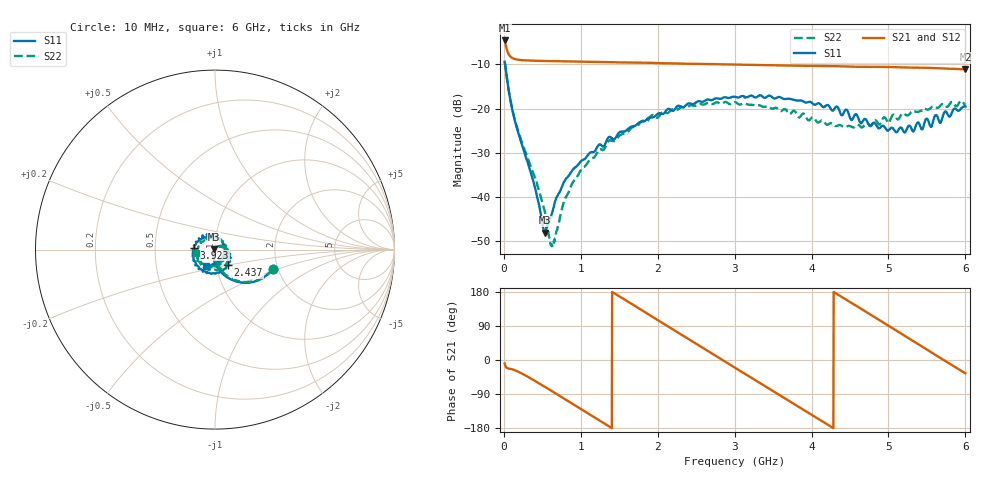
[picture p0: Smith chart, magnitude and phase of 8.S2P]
!Agilent Technologies,E5071C,MY46316741,A.11.02
!Date: Thu Jul 30 16:12:56 2020
!Data & Calibration Information:
!Freq	S11:SOLT4(ON)	S21:SOLT4(ON)	S12:SOLT4(ON)	S22:SOLT4(ON)
!PortZ  Port1:50+j0  Port2:50+j0
!Above PortZ is port z conversion or system Z0 setting when saving the data.
!When reading, reference impedance value at option line is always used.
# Hz S dB R 50
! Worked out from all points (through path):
!   1561 points, 10 MHz to 6 GHz, reference 50 ohm
!   highest |S21| = -4.55 dB at 10 MHz (marker M1); lowest = -11.1 dB at 6 GHz (marker M2)
!   group delay of S21, straight-line fit = 347 ps
!   lowest |S11| = -48.2 dB at 536 MHz (marker M3), VSWR 1.01, Z = 49.6 + j0.164 ohm
!   |S11| at or under -10 dB: 16.33 MHz to end of sweep
!   |S22| runs from -51.2 to -9.3 dB; largest |S21 - S12| = 0.0045
!   S11 on the Smith chart (normalised r, x): 10 MHz: 1.88, -0.46; 2.437 GHz: 1.14, -0.20; 3.923 GHz: 0.79, +0.02; 6 GHz: 0.89, -0.17
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1e7  -9.37 -18.6  -4.55 -9.1  -4.55 -9.1  -9.34 -18.2
5.991667e7  -15.52 -66.5  -7.59 -22.5  -7.59 -22.5  -15.48 -63.7
1.136731e8  -20.59 -83.8  -8.57 -24.9  -8.56 -24.9  -20.48 -78.3
3.786154e8  -36.22 -125.3  -9.15 -52.1  -9.14 -52.2  -34.53 -95.8
5.360449e8  -48.19 154.9  -9.21 -71.1  -9.21 -71.2  -43.60 -84.3
5.974808e8  -45.26 108.7  -9.23 -78.7  -9.23 -78.8  -50.08 -60.3
6.358782e8  -43.14 88.3  -9.25 -83.4  -9.24 -83.5  -50.97 -23.1
7.894679e8  -36.49 62.1  -9.29 -102.5  -9.29 -102.7  -40.59 42.0
1.012173e9  -31.80 46.9  -9.35 -130.4  -9.35 -130.6  -33.70 41.9
1.488301e9  -25.67 16.2  -9.53 169.7  -9.52 169.4  -26.42 15.0
2.006667e9  -21.13 -17.1  -9.69 104.5  -9.69 104.4  -21.99 -24.8
2.436718e9  -18.91 -50.6  -9.84 50.8  -9.84 50.4  -19.24 -62.7
2.724699e9  -17.91 -77.0  -9.93 14.8  -9.92 14.4  -18.92 -92.7
3.005e9  -17.34 -99.8  -10.01 -20.4  -10.01 -20.8  -18.54 -120.8
3.473449e9  -17.22 -141.4  -10.19 -78.8  -10.17 -79.3  -19.96 -171.7
3.922699e9  -18.64 174.7  -10.32 -134.8  -10.31 -135.4  -21.69 133.8
4.007173e9  -18.75 167.8  -10.35 -145.3  -10.33 -145.9  -22.02 116.0
4.448744e9  -20.23 116.8  -10.46 159.3  -10.46 158.5  -24.12 44.9
4.517859e9  -22.60 109.4  -10.50 150.7  -10.50 150.0  -24.13 36.3
5.001667e9  -24.94 33.0  -10.57 90.1  -10.57 89.3  -23.31 -43.6
5.531551e9  -23.40 -54.8  -10.78 23.4  -10.77 22.6  -20.14 -113.4
6e9  -19.54 -118.0  -11.10 -35.1  -11.08 -36.0  -19.26 -168.5
